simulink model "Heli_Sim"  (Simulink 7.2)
settings: Solver=ode45  SolverMode=SingleTasking  StartTime=0.0  StopTime=10.0  RelTol=1e-3  AbsTol=1e-6
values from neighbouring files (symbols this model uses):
  c_GR = 0.028    [Helipar.m]
  c_GS = 0.0091    [Helipar.m]
  c_MR = 0.028    [Helipar.m]
  c_MS = 0.0091    [Helipar.m]
  c_muH = 5e-3    (= 0.005)    [Helipar.m]
  c_muR = 1e-5    (= 1e-05)    [Helipar.m]
  c_muS = 1e-5    (= 1e-05)    [Helipar.m]
  c_muV = 5e-2    (= 0.05)    [Helipar.m]
  g = 9.81    [Helipar.m]
  i_max = 10    [Helipar.m]
  k_FR = 2.4e-5    (= 2.4e-05)    [Helipar.m]
  k_FS = 2.7e-6    (= 2.7e-06)    [Helipar.m]
  k_messH = 3.29    [Helipar.m]
  k_messV = 3.36    [Helipar.m]
  k_MR = 1e-6    (= 1e-06)    [Helipar.m]
  k_MS = 1e-7    (= 1e-07)    [Helipar.m]
  m_G = 1.19    [Helipar.m]
  phi_maxH = 60*pi/180    (= 1.0471975512)    [Helipar.m]
  phi_maxV = 170*pi/180    (= 2.96705972839)    [Helipar.m]
  phi_minH = -phi_maxH    (= -1.0471975512)    [Helipar.m]
  phi_minV = -phi_maxV    (= -2.96705972839)    [Helipar.m]
  phistart_H = 0    [Helipar.m]
  phistart_V = 0    [Helipar.m]
  r_H = 0.0157    [Helipar.m]
  r_R = 0.1995    [Helipar.m]
  R_R = 0.9    [Helipar.m]
  r_S = 0.1743    [Helipar.m]
  R_S = 1.2    [Helipar.m]
  r_V = 0.0298    [Helipar.m]
  theta_H = 0.027    [Helipar.m]
  theta_R = 4.8e-4    (= 0.00048)    [Helipar.m]
  theta_S = 3.2e-5    (= 3.2e-05)    [Helipar.m]
  theta_V1 = 0.027    [Helipar.m]
  theta_V2 = 2.0e-4    (= 0.0002)    [Helipar.m]
  theta_zyl = 1e-5    (= 1e-05)    [Helipar.m]
  u_max_phi = 16    [Helipar.m]
  u_max_psi = 8    [Helipar.m]

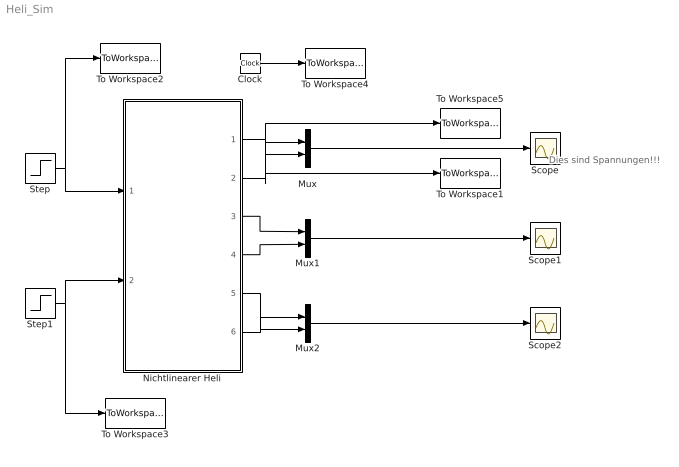
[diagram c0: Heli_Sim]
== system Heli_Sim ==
  note: Dies sind Spannungen!!!
  Clock : Clock
  Mux : Mux  Inputs=2
  Mux1 : Mux  Inputs=2
  Mux2 : Mux  Inputs=2
  Nichtlinearer Heli : Subsystem
  Scope : Scope
  Scope1 : Scope
  Scope2 : Scope
  Step : Step  After=10  SampleTime=0
  Step1 : Step  Time=5  After=8  SampleTime=0
  To Workspace1 : ToWorkspace  VariableName=Upsi  SampleTime=-1  SaveFormat=Array
  To Workspace2 : ToWorkspace  VariableName=Usphi  SampleTime=-1  SaveFormat=Array
  To Workspace3 : ToWorkspace  VariableName=Uspsi  SampleTime=-1  SaveFormat=Array
  To Workspace4 : ToWorkspace  VariableName=t  SampleTime=-1  SaveFormat=Array
  To Workspace5 : ToWorkspace  VariableName=Uphi  SampleTime=-1  SaveFormat=Array
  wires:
  Clock/1 -> To Workspace4/1
  Step1/1 -> To Workspace3/1, Nichtlinearer Heli/2(u_S)
  Step/1 -> To Workspace2/1, Nichtlinearer Heli/1(u_R)
  Nichtlinearer Heli/1(U_phi_H) -> To Workspace5/1, Mux/1
  Nichtlinearer Heli/2(U_phi_V) -> To Workspace1/1, Mux/2
  Mux/1 -> Scope/1
  Nichtlinearer Heli/3(omega_R) -> Mux1/1
  Nichtlinearer Heli/4(omega_S) -> Mux1/2
  Nichtlinearer Heli/5(i_R) -> Mux2/1
  Nichtlinearer Heli/6(i_S) -> Mux2/2
  Mux1/1 -> Scope1/1
  Mux2/1 -> Scope2/1

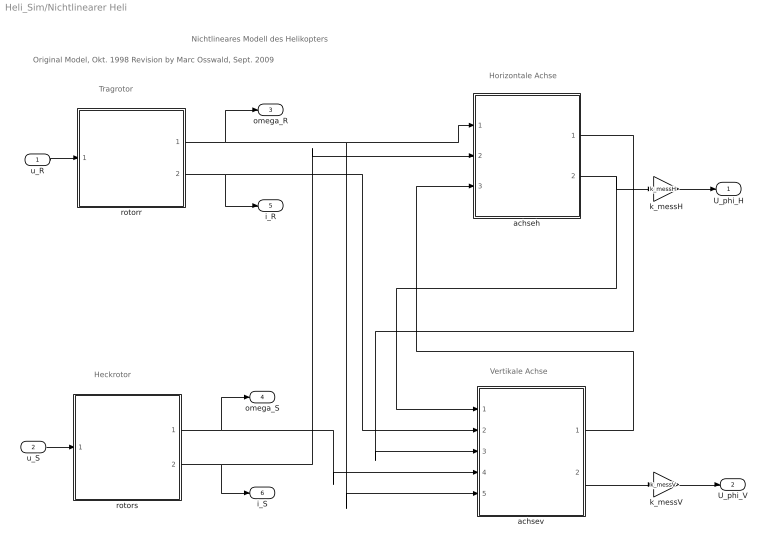
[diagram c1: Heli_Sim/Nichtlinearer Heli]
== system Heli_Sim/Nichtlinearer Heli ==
  note: Vertikale Achse
  note: Horizontale Achse
  note: Heckrotor
  note: Tragrotor
  note: Nichtlineares Modell des Helikopters
  note: Original Model, Okt. 1998 Revision by Marc Osswald, Sept. 2009
  u_R : Inport  OutDataType=sfix(16)  OutScaling=2^0
  u_S : Inport  Port=2  OutDataType=sfix(16)  OutScaling=2^0
  achseh : Subsystem
  achsev : Subsystem
  k_messH : Gain  Gain=k_messH  ParameterDataType=sfix(16)  ParameterScaling=2^0  OutDataType=sfix(16)  OutScaling=2^0
  k_messV : Gain  Gain=k_messV  ParameterDataType=sfix(16)  ParameterScaling=2^0  OutDataType=sfix(16)  OutScaling=2^0
  rotorr : Subsystem
  rotors : Subsystem
  U_phi_H : Outport  InitialOutput=0
  U_phi_V : Outport  Port=2  InitialOutput=0
  omega_R : Outport  Port=3  OutDataType=sfix(16)  OutScaling=2^0
  omega_S : Outport  Port=4  OutDataType=sfix(16)  OutScaling=2^0
  i_R : Outport  Port=5  OutDataType=sfix(16)  OutScaling=2^0
  i_S : Outport  Port=6  OutDataType=sfix(16)  OutScaling=2^0
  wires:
  u_R/1 -> rotorr/1(u_R)
  u_S/1 -> rotors/1(u_s)
  achsev/2(phi_V) -> k_messV/1
  k_messV/1 -> U_phi_V/1
  k_messH/1 -> U_phi_H/1
  achseh/2(phi_H) -> achsev/1(phi_H), k_messH/1
  achseh/1(omega_H) -> achsev/3(omega_H)
  achsev/1(omega_V) -> achseh/3(omega_V)
  rotors/1(omega_S) -> achsev/4(omega_S), omega_S/1
  rotors/2(i_S) -> achseh/2(i_S), i_S/1
  rotorr/2(i_r) -> achsev/2(i_R), i_R/1
  rotorr/1(omega_R) -> achsev/5(omega_R), achseh/1(omega_R), omega_R/1

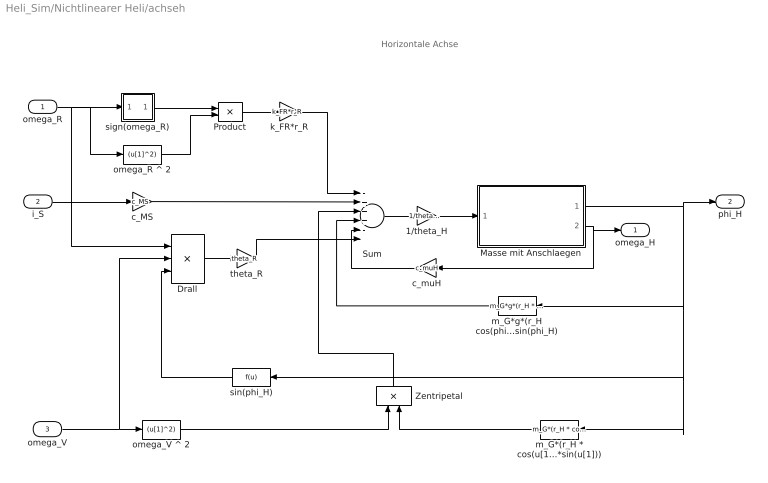
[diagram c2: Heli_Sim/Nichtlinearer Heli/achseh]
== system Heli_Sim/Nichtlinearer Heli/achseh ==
  note: Horizontale Achse
  omega_R : Inport  OutDataType=sfix(16)  OutScaling=2^0
  i_S : Inport  Port=2  OutDataType=sfix(16)  OutScaling=2^0
  omega_V : Inport  Port=3  OutDataType=sfix(16)  OutScaling=2^0
  1/theta_H : Gain  Gain=1/theta_H  ParameterDataType=sfix(16)  ParameterScaling=2^0  OutDataType=sfix(16)  OutScaling=2^0
  Drall : Product  Inputs=3  OutDataType=sfix(16)  OutScaling=2^0
  Masse mit Anschlaegen : Subsystem
  Product : Product  OutDataType=sfix(16)  OutScaling=2^0
  Sum : Sum  Inputs=-+++-+  OutDataType=sfix(16)  OutScaling=2^0
  Zentripetal : Product  Orientation=up  OutDataType=sfix(16)  OutScaling=2^0
  c_MS : Gain  Gain=c_MS  ParameterDataType=sfix(16)  ParameterScaling=2^0  OutDataType=sfix(16)  OutScaling=2^0
  c_muH : Gain  Orientation=left  Gain=c_muH  ParameterDataType=sfix(16)  ParameterScaling=2^0  OutDataType=sfix(16)  OutScaling=2^0
  k_FR*r_R : Gain  Gain=k_FR*r_R  ParameterDataType=sfix(16)  ParameterScaling=2^0  OutDataType=sfix(16)  OutScaling=2^0
  m_G*(r_H * cos(u[1]) + r_V * sin(u[1]))*(r_V*cos(u[1])-r_H*sin(u[1])) : Fcn  Orientation=left  Expr=m_G*(r_H * cos(u[1]) + r_V * sin(u[1]))*(r_V*cos(u[1])-r_H*sin(u[1]))
  m_G*g*(r_H cos(phi_H) + r_V sin(phi_H) : Fcn  Orientation=left  Expr=m_G*g*(r_H * cos(u[1]) + r_V * sin(u[1]))
  omega_R ^ 2 : Fcn  Expr=(u[1]^2)
  omega_V ^ 2 : Fcn  Expr=(u[1]^2)
  sign(omega_R) : Subsystem
  sin(phi_H) : Fcn  Orientation=left
  theta_R : Gain  Gain=theta_R  ParameterDataType=sfix(16)  ParameterScaling=2^0  OutDataType=sfix(16)  OutScaling=2^0
  omega_H : Outport  InitialOutput=0
  phi_H : Outport  Port=2  InitialOutput=0
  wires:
  m_G*(r_H * cos(u[1]) + r_V * sin(u[1]))*(r_V*cos(u[1])-r_H*sin(u[1]))/1 -> Zentripetal/2
  Zentripetal/1 -> Sum/3
  theta_R/1 -> Sum/6
  Drall/1 -> theta_R/1
  sin(phi_H)/1 -> Drall/3
  m_G*g*(r_H cos(phi_H) + r_V sin(phi_H)/1 -> Sum/4
  k_FR*r_R/1 -> Sum/1
  omega_V/1 -> Drall/2, omega_V ^ 2/1
  omega_R/1 -> Drall/1, omega_R ^ 2/1, sign(omega_R)/1(in_1)
  sign(omega_R)/1(out_1) -> Product/1
  omega_V ^ 2/1 -> Zentripetal/1
  Masse mit Anschlaegen/1(Position) -> m_G*(r_H * cos(u[1]) + r_V * sin(u[1]))*(r_V*cos(u[1])-r_H*sin(u[1]))/1, sin(phi_H)/1, m_G*g*(r_H cos(phi_H) + r_V sin(phi_H)/1, phi_H/1
  Masse mit Anschlaegen/2(Geschwindigkeit) -> omega_H/1, c_muH/1
  c_muH/1 -> Sum/5
  1/theta_H/1 -> Masse mit Anschlaegen/1(Beschleunigung)
  Sum/1 -> 1/theta_H/1
  i_S/1 -> c_MS/1
  Product/1 -> k_FR*r_R/1
  omega_R ^ 2/1 -> Product/2
  c_MS/1 -> Sum/2

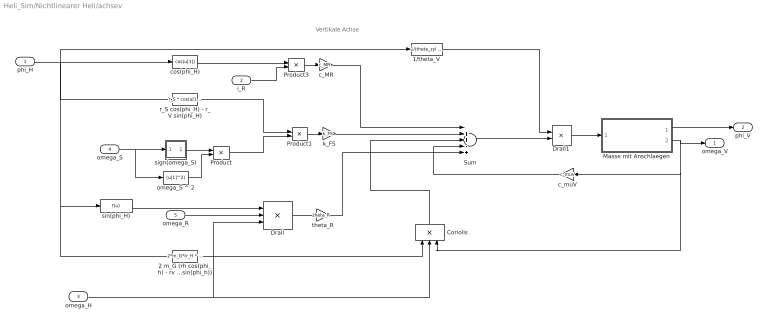
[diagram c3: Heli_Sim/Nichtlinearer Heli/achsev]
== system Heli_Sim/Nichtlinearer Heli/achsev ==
  note: Vertikale Achse
  phi_H : Inport  OutDataType=sfix(16)  OutScaling=2^0
  i_R : Inport  Port=2  OutDataType=sfix(16)  OutScaling=2^0
  omega_H : Inport  Port=3  OutDataType=sfix(16)  OutScaling=2^0
  omega_S : Inport  Port=4  OutDataType=sfix(16)  OutScaling=2^0
  omega_R : Inport  Port=5  OutDataType=sfix(16)  OutScaling=2^0
  1/theta_V : Fcn  Expr=1/(theta_zyl + theta_V1*cos(u[1])^2 + theta_V2*sin(u[1])^2 + m_G*(r_H*cos(u[1])-r_V*sin(u[1]))^2)
  2 m_G (rh cos(phi_h) - rv sin(phi_h))*(rv cos(phi_h) + rh sin(phi_h)) : Fcn  Expr=2*m_G*(r_H * cos(u[1]) + r_V * sin(u[1]))*(r_V * cos(u[1]) - r_H * sin(u[1]))
  Coriolis : Product  Orientation=up  Inputs=3  OutDataType=sfix(16)  OutScaling=2^0
  Drall : Product  Inputs=3  OutDataType=sfix(16)  OutScaling=2^0
  Drall1 : Product  OutDataType=sfix(16)  OutScaling=2^0
  Masse mit Anschlaegen : Subsystem
  Product : Product  OutDataType=sfix(16)  OutScaling=2^0
  Product1 : Product  OutDataType=sfix(16)  OutScaling=2^0
  Product3 : Product  OutDataType=sfix(16)  OutScaling=2^0
  Sum : Sum  Inputs=-++-+  OutDataType=sfix(16)  OutScaling=2^0
  c_MR : Gain  Gain=c_MR  ParameterDataType=sfix(16)  ParameterScaling=2^0  OutDataType=sfix(16)  OutScaling=2^0
  c_muV : Gain  Orientation=left  Gain=c_muV  ParameterDataType=sfix(16)  ParameterScaling=2^0  OutDataType=sfix(16)  OutScaling=2^0
  cos(phi_H) : Fcn  Expr=cos(u[1])
  k_FS : Gain  Gain=k_FS  ParameterDataType=sfix(16)  ParameterScaling=2^0  OutDataType=sfix(16)  OutScaling=2^0
  omega_S ^ 2 : Fcn  Expr=(u[1]^2)
  r_S cos(phi_H) - r_V sin(phi_H) : Fcn  Expr=r_S * cos(u[1]) - r_V * sin(u[1])
  sign(omega_S) : Subsystem
  sin(phi_H) : Fcn
  theta_R : Gain  Gain=theta_R  ParameterDataType=sfix(16)  ParameterScaling=2^0  OutDataType=sfix(16)  OutScaling=2^0
  omega_V : Outport  InitialOutput=0
  phi_V : Outport  Port=2  InitialOutput=0
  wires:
  1/theta_V/1 -> Drall1/1
  Masse mit Anschlaegen/2(Geschwindigkeit) -> Coriolis/3, c_muV/1, omega_V/1
  Drall1/1 -> Masse mit Anschlaegen/1(Beschleunigung)
  Masse mit Anschlaegen/1(Position) -> phi_V/1
  Sum/1 -> Drall1/2
  2 m_G (rh cos(phi_h) - rv sin(phi_h))*(rv cos(phi_h) + rh sin(phi_h))/1 -> Coriolis/1
  omega_H/1 -> Drall/3, Coriolis/2
  Coriolis/1 -> Sum/3
  omega_S/1 -> omega_S ^ 2/1, sign(omega_S)/1(in_1)
  phi_H/1 -> 1/theta_V/1, sin(phi_H)/1, 2 m_G (rh cos(phi_h) - rv sin(phi_h))*(rv cos(phi_h) + rh sin(phi_h))/1, r_S cos(phi_H) - r_V sin(phi_H)/1, cos(phi_H)/1
  cos(phi_H)/1 -> Product3/1
  omega_R/1 -> Drall/2
  sin(phi_H)/1 -> Drall/1
  Drall/1 -> theta_R/1
  sign(omega_S)/1(out_1) -> Product/1
  omega_S ^ 2/1 -> Product/2
  Product/1 -> Product1/2
  i_R/1 -> Product3/2
  Product1/1 -> k_FS/1
  r_S cos(phi_H) - r_V sin(phi_H)/1 -> Product1/1
  Product3/1 -> c_MR/1
  c_MR/1 -> Sum/1
  c_muV/1 -> Sum/4
  k_FS/1 -> Sum/2
  theta_R/1 -> Sum/5

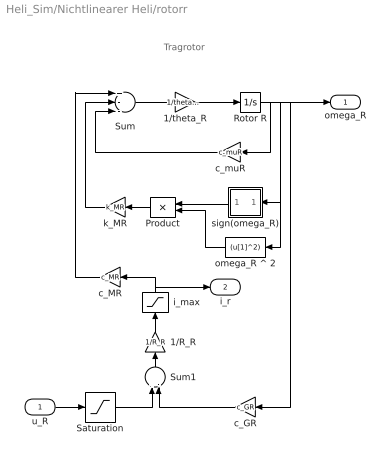
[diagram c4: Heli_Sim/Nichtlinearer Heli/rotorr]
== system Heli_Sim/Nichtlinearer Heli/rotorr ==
  note: Tragrotor
  u_R : Inport  OutDataType=sfix(16)  OutScaling=2^0
  1/R_R : Gain  Orientation=up  Gain=1/R_R  ParameterDataType=sfix(16)  ParameterScaling=2^0  OutDataType=sfix(16)  OutScaling=2^0
  1/theta_R : Gain  Gain=1/theta_R  ParameterDataType=sfix(16)  ParameterScaling=2^0  OutDataType=sfix(16)  OutScaling=2^0
  Product : Product  Orientation=left  OutDataType=sfix(16)  OutScaling=2^0
  Rotor R : Integrator
  Saturation : Saturate  UpperLimit=u_max_phi  LowerLimit=-u_max_phi
  Sum : Sum  Inputs=+--  OutDataType=sfix(16)  OutScaling=2^0
  Sum1 : Sum  Orientation=up  Inputs=+-  OutDataType=sfix(16)  OutScaling=2^0
  c_GR : Gain  Orientation=left  Gain=c_GR  ParameterDataType=sfix(16)  ParameterScaling=2^0  OutDataType=sfix(16)  OutScaling=2^0
  c_MR : Gain  Orientation=left  Gain=c_MR  ParameterDataType=sfix(16)  ParameterScaling=2^0  OutDataType=sfix(16)  OutScaling=2^0
  c_muR : Gain  Orientation=left  Gain=c_muR  ParameterDataType=sfix(16)  ParameterScaling=2^0  OutDataType=sfix(16)  OutScaling=2^0
  i_max : Saturate  Orientation=up  UpperLimit=i_max  LowerLimit=-i_max
  k_MR : Gain  Orientation=left  Gain=k_MR  ParameterDataType=sfix(16)  ParameterScaling=2^0  OutDataType=sfix(16)  OutScaling=2^0
  omega_R ^ 2 : Fcn  Orientation=left  Expr=(u[1]^2)
  sign(omega_R) : Subsystem  Orientation=left
  omega_R : Outport  InitialOutput=0
  i_r : Outport  Port=2  InitialOutput=0
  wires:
  Saturation/1 -> Sum1/1
  u_R/1 -> Saturation/1
  i_max/1 -> i_r/1, c_MR/1
  1/R_R/1 -> i_max/1
  c_MR/1 -> Sum/1
  Sum1/1 -> 1/R_R/1
  c_GR/1 -> Sum1/2
  Product/1 -> k_MR/1
  omega_R ^ 2/1 -> Product/2
  sign(omega_R)/1(out_1) -> Product/1
  k_MR/1 -> Sum/2
  Rotor R/1 -> omega_R/1, c_GR/1, omega_R ^ 2/1, sign(omega_R)/1(in_1), c_muR/1
  c_muR/1 -> Sum/3
  1/theta_R/1 -> Rotor R/1
  Sum/1 -> 1/theta_R/1

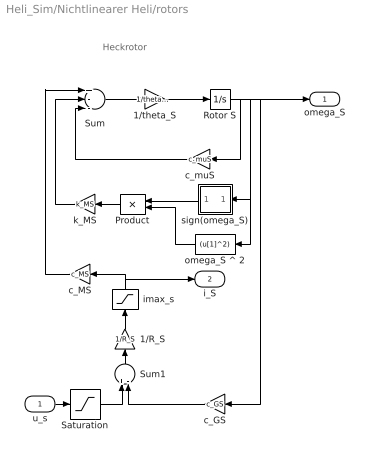
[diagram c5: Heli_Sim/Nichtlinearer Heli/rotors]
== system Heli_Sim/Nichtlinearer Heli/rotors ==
  note: Heckrotor
  u_s : Inport  OutDataType=sfix(16)  OutScaling=2^0
  1/R_S : Gain  Orientation=up  Gain=1/R_S  ParameterDataType=sfix(16)  ParameterScaling=2^0  OutDataType=sfix(16)  OutScaling=2^0
  1/theta_S : Gain  Gain=1/theta_S  ParameterDataType=sfix(16)  ParameterScaling=2^0  OutDataType=sfix(16)  OutScaling=2^0
  Product : Product  Orientation=left  OutDataType=sfix(16)  OutScaling=2^0
  Rotor S : Integrator
  Saturation : Saturate  UpperLimit=u_max_psi  LowerLimit=-u_max_psi
  Sum : Sum  Inputs=+--  OutDataType=sfix(16)  OutScaling=2^0
  Sum1 : Sum  Orientation=up  Inputs=+-  OutDataType=sfix(16)  OutScaling=2^0
  c_GS : Gain  Orientation=left  Gain=c_GS  ParameterDataType=sfix(16)  ParameterScaling=2^0  OutDataType=sfix(16)  OutScaling=2^0
  c_MS : Gain  Orientation=left  Gain=c_MS  ParameterDataType=sfix(16)  ParameterScaling=2^0  OutDataType=sfix(16)  OutScaling=2^0
  c_muS : Gain  Orientation=left  Gain=c_muS  ParameterDataType=sfix(16)  ParameterScaling=2^0  OutDataType=sfix(16)  OutScaling=2^0
  imax_s : Saturate  Orientation=up  UpperLimit=i_max  LowerLimit=-i_max
  k_MS : Gain  Orientation=left  Gain=k_MS  ParameterDataType=sfix(16)  ParameterScaling=2^0  OutDataType=sfix(16)  OutScaling=2^0
  omega_S ^ 2 : Fcn  Orientation=left  Expr=(u[1]^2)
  sign(omega_S) : Subsystem  Orientation=left
  omega_S : Outport  InitialOutput=0
  i_S : Outport  Port=2  InitialOutput=0
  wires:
  Saturation/1 -> Sum1/1
  u_s/1 -> Saturation/1
  imax_s/1 -> i_S/1, c_MS/1
  1/R_S/1 -> imax_s/1
  c_MS/1 -> Sum/1
  Sum1/1 -> 1/R_S/1
  c_GS/1 -> Sum1/2
  Product/1 -> k_MS/1
  omega_S ^ 2/1 -> Product/2
  sign(omega_S)/1(out_1) -> Product/1
  k_MS/1 -> Sum/2
  Rotor S/1 -> omega_S/1, c_GS/1, omega_S ^ 2/1, sign(omega_S)/1(in_1), c_muS/1
  c_muS/1 -> Sum/3
  1/theta_S/1 -> Rotor S/1
  Sum/1 -> 1/theta_S/1

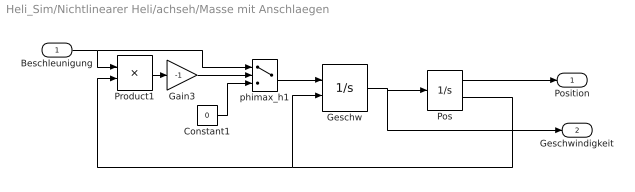
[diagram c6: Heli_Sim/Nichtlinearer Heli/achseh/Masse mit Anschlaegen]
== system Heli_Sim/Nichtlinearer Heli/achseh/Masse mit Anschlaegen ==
  Beschleunigung : Inport  OutDataType=sfix(16)  OutScaling=2^0
  Constant1 : Constant  Value=0  OutDataType=sfix(16)  OutScaling=2^0
  Gain3 : Gain  Gain=-1  ParameterDataType=sfix(16)  ParameterScaling=2^0  OutDataType=sfix(16)  OutScaling=2^0
  Geschw : Integrator  ExternalReset=either
  Pos : Integrator  InitialCondition=phistart_H  LimitOutput=on  UpperSaturationLimit=phi_maxH  LowerSaturationLimit=phi_minH  ShowSaturationPort=on
  Product1 : Product  OutDataType=sfix(16)  OutScaling=2^0
  phimax_h1 : Switch
  Position : Outport  InitialOutput=0
  Geschwindigkeit : Outport  Port=2  InitialOutput=0
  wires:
  Beschleunigung/1 -> Product1/1, phimax_h1/1
  Product1/1 -> Gain3/1
  Gain3/1 -> phimax_h1/2
  Constant1/1 -> phimax_h1/3
  phimax_h1/1 -> Geschw/1
  Geschw/1 -> Geschwindigkeit/1, Pos/1
  Pos/1 -> Position/1
  Pos/2 -> Product1/2, Geschw/2

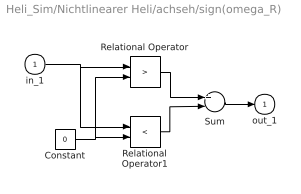
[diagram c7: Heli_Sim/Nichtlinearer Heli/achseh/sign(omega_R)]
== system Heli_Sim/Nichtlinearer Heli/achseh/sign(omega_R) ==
  in_1 : Inport  OutDataType=sfix(16)  OutScaling=2^0
  Constant : Constant  Value=0  OutDataType=sfix(16)  OutScaling=2^0
  Relational Operator : RelationalOperator  Operator=>
  Relational Operator1 : RelationalOperator  Operator=<
  Sum : Sum  Inputs=+-  OutDataType=sfix(16)  OutScaling=2^0
  out_1 : Outport  InitialOutput=0
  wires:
  in_1/1 -> Relational Operator1/1, Relational Operator/1
  Constant/1 -> Relational Operator/2, Relational Operator1/2
  Relational Operator1/1 -> Sum/2
  Relational Operator/1 -> Sum/1
  Sum/1 -> out_1/1

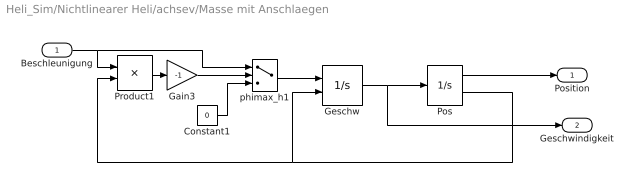
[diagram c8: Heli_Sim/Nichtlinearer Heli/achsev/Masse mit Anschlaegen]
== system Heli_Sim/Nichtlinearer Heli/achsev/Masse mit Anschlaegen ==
  Beschleunigung : Inport  OutDataType=sfix(16)  OutScaling=2^0
  Constant1 : Constant  Value=0  OutDataType=sfix(16)  OutScaling=2^0
  Gain3 : Gain  Gain=-1  ParameterDataType=sfix(16)  ParameterScaling=2^0  OutDataType=sfix(16)  OutScaling=2^0
  Geschw : Integrator  ExternalReset=either
  Pos : Integrator  InitialCondition=phistart_V  LimitOutput=on  UpperSaturationLimit=phi_maxV  LowerSaturationLimit=phi_minV  ShowSaturationPort=on
  Product1 : Product  OutDataType=sfix(16)  OutScaling=2^0
  phimax_h1 : Switch
  Position : Outport  InitialOutput=0
  Geschwindigkeit : Outport  Port=2  InitialOutput=0
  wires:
  Geschw/1 -> Geschwindigkeit/1, Pos/1
  Pos/1 -> Position/1
  Beschleunigung/1 -> Product1/1, phimax_h1/1
  Product1/1 -> Gain3/1
  Gain3/1 -> phimax_h1/2
  Constant1/1 -> phimax_h1/3
  phimax_h1/1 -> Geschw/1
  Pos/2 -> Product1/2, Geschw/2

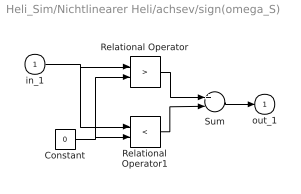
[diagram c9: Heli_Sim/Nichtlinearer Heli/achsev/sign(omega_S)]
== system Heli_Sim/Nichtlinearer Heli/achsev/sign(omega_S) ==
  in_1 : Inport  OutDataType=sfix(16)  OutScaling=2^0
  Constant : Constant  Value=0  OutDataType=sfix(16)  OutScaling=2^0
  Relational Operator : RelationalOperator  Operator=>
  Relational Operator1 : RelationalOperator  Operator=<
  Sum : Sum  Inputs=+-  OutDataType=sfix(16)  OutScaling=2^0
  out_1 : Outport  InitialOutput=0
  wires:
  in_1/1 -> Relational Operator1/1, Relational Operator/1
  Constant/1 -> Relational Operator/2, Relational Operator1/2
  Relational Operator1/1 -> Sum/2
  Relational Operator/1 -> Sum/1
  Sum/1 -> out_1/1

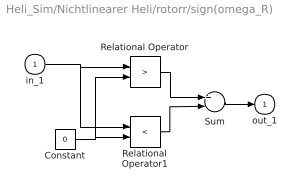
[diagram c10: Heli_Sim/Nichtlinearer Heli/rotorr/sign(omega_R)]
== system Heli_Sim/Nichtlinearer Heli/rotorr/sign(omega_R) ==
  in_1 : Inport  OutDataType=sfix(16)  OutScaling=2^0
  Constant : Constant  Value=0  OutDataType=sfix(16)  OutScaling=2^0
  Relational Operator : RelationalOperator  Operator=>
  Relational Operator1 : RelationalOperator  Operator=<
  Sum : Sum  Inputs=+-  OutDataType=sfix(16)  OutScaling=2^0
  out_1 : Outport  InitialOutput=0
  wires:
  Sum/1 -> out_1/1
  Relational Operator/1 -> Sum/1
  Relational Operator1/1 -> Sum/2
  Constant/1 -> Relational Operator/2, Relational Operator1/2
  in_1/1 -> Relational Operator1/1, Relational Operator/1

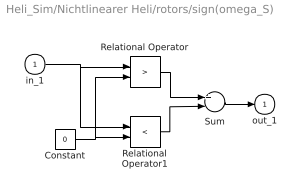
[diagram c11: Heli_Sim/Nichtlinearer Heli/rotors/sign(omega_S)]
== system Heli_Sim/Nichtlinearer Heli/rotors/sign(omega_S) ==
  in_1 : Inport  OutDataType=sfix(16)  OutScaling=2^0
  Constant : Constant  Value=0  OutDataType=sfix(16)  OutScaling=2^0
  Relational Operator : RelationalOperator  Operator=>
  Relational Operator1 : RelationalOperator  Operator=<
  Sum : Sum  Inputs=+-  OutDataType=sfix(16)  OutScaling=2^0
  out_1 : Outport  InitialOutput=0
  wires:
  Sum/1 -> out_1/1
  Relational Operator/1 -> Sum/1
  Relational Operator1/1 -> Sum/2
  Constant/1 -> Relational Operator/2, Relational Operator1/2
  in_1/1 -> Relational Operator1/1, Relational Operator/1
